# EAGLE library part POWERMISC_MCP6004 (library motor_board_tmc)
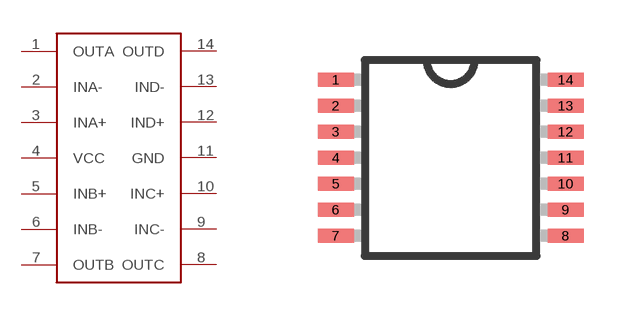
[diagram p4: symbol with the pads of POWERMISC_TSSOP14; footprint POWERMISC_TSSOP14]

Designator prefix U

## POWERMISC_MCP6004  [POWERMISC_TSSOP14]
1  OUTA
2  INA-
3  INA+
4  VCC
5  INB+
6  INB-
7  OUTB
8  OUTC
9  INC-
10  INC+
11  GND
12  IND+
13  IND-
14  OUTD

## Footprint POWERMISC_TSSOP14 (pad centres in mm)
14-Lead Thin Shrink Small Outline Package [TSSOP] Source: Analog Devices .. 780914713ADD8704_0.pdf
smd 0.9 x 0.35: 1 -2.875,1.95; 2 -2.875,1.3; 3 -2.875,0.65; 4 -2.875,0; 5 -2.875,-0.65; 6 -2.875,-1.3; 7 -2.875,-1.95; 8 2.875,-1.95; 9 2.875,-1.3; 10 2.875,-0.65; 11 2.875,0; 12 2.875,0.65; 13 2.875,1.3; 14 2.875,1.95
